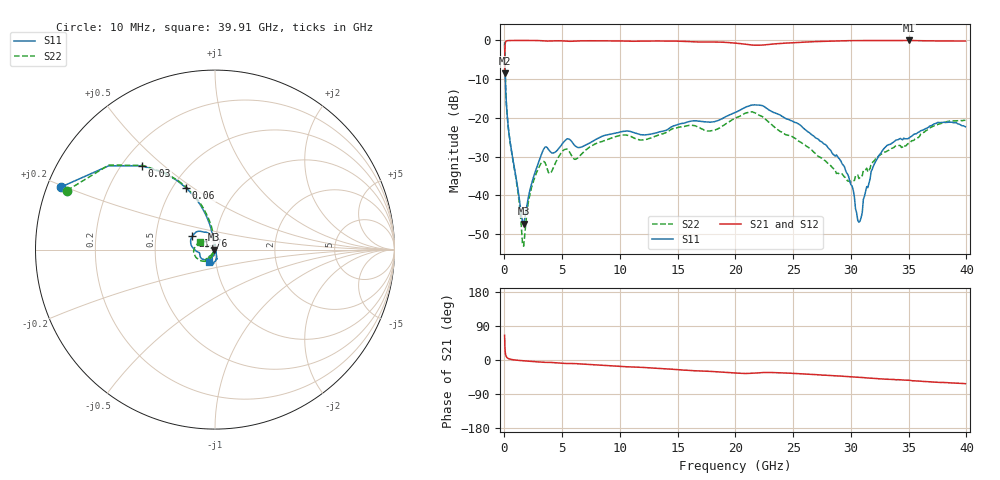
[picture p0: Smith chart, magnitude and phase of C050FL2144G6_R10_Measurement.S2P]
! Data measured by Modelithics Inc.  support@modelithics.com  813-866-6335  Tampa FL USA June 2025
! PPI-050FL-0R28-280-G6_0p28uH measured on 10-mil thick RO4350B board, mounted in 2-port shunt configuration on a 50-ohm transmission line
# Hz S MA R 50
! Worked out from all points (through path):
!   429 points, 10 MHz to 39.91 GHz, reference 50 ohm
!   highest |S21| = -0.04 dB at 35.06 GHz (marker M1); lowest = -8.5 dB at 10 MHz (marker M2)
!   group delay of S21, straight-line fit = 4.52 ps
!   lowest |S11| = -47.3 dB at 1.659 GHz (marker M3), VSWR 1.01, Z = 49.6 - j0.0893 ohm
!   |S11| at or under -10 dB: 74.46 MHz to end of sweep
!   |S22| runs from -53.1 to -1.0 dB; largest |S21 - S12| = 0.025
!   S11 on the Smith chart (normalised r, x): 10 MHz: 0.04, +0.20; 30 MHz: 0.28, +0.42; 60 MHz: 0.58, +0.47; 21.76 GHz: 0.77, +0.12; 39.91 GHz: 0.93, -0.13
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1e7  0.9266 157.9  0.3748 65.1  0.3746 65.1  0.8883 158.2
3e7  0.6194 131.1  0.7558 38.2  0.7557 38.2  0.6201 130.8
6e7  0.3791 115.1  0.9078 22.2  0.9078 22.2  0.3786 114.4
2e8  0.125 101.0  0.9851 6.9  0.985 6.9  0.1247 98.5
1.659243e9  0.004299 -167.9  0.9956 -2.1  0.9956 -2.1  0.002209 -170.6
2.241776e9  0.01236 -107.2  0.9954 -3.5  0.9953 -3.5  0.01093 -113.2
3.115575e9  0.03121 -99.8  0.99 -5.6  0.9901 -5.5  0.02519 -123.2
3.989374e9  0.03627 -124.8  0.9826 -6.4  0.9825 -6.4  0.01933 -126.6
5.445706e9  0.05357 -121.4  0.9736 -9.3  0.9737 -9.3  0.03915 -132.5
6.70786e9  0.04216 -116.1  0.9845 -10.6  0.9843 -10.6  0.03445 -115.3
9.91179e9  0.06486 -112.4  0.9813 -16.8  0.9812 -16.6  0.0587 -120.6
1.340699e10  0.0659 -128.0  0.9794 -22.3  0.9794 -22.4  0.0605 -117.0
2.000902e10  0.1179 177.5  0.9191 -34.5  0.919 -34.6  0.09962 -141.4
2.175662e10  0.1468 149.6  0.8644 -34.4  0.8644 -34.2  0.1148 175.5
2.670815e10  0.05915 94.3  0.9597 -38.0  0.9595 -38.0  0.03706 98.4
2.923246e10  0.02561 85.9  0.9839 -42.8  0.9839 -42.8  0.01887 106.1
3.068879e10  0.004491 23.3  0.992 -45.8  0.9919 -45.9  0.01645 140.1
3.195095e10  0.02397 -73.0  0.9919 -48.3  0.9918 -48.5  0.02729 164.0
3.331019e10  0.04525 -79.4  0.9912 -50.8  0.9912 -51.0  0.03817 165.3
3.505779e10  0.05522 -82.3  0.9957 -53.6  0.9957 -54.9  0.04685 162.2
3.748501e10  0.08682 -99.3  0.9806 -58.5  0.9806 -58.4  0.08168 161.5
3.991223e10  0.07663 -115.9  0.9785 -62.5  0.9782 -62.0  0.09282 153.0
